[IBIS Ver]   3.2
[File Name]   sprm039d.ibs
[File Rev]   0.6
[Date]   April 12, 2004
[Source]   File Originated at Texas Instruments
[Disclaimer]   Please be aware that in the absence of a written agreement
|   Texas Instruments(TI) assumes no liability for:
|   (1) The accuracy of the IBIS models provided to your company
|   (2) The proper functioning of these Models in your design
|   or for any resulting applications;or
|   (3) Infringement of patents,copyrights, or intellectual
|   property rights resulting from your use of these models.
|   TI provides IBIS Models as a service to our customers and
|   therefore reserves the right to limit distribution of the
|   Models.
[Copyright]   Property of Texas Instruments Incorporated.
|   Unauthorized reproduction and/or distribution is strictly
|   prohibited.
|   This product is protected under copyright law and trade
|   secret law as an unpublished work.
|   Created 1999,(C) Copyright 1999-2000,
|   Texas Instruments Incorporated., All Rights Reserved.
|   These commodities are under the U.S.
|   Government distribution license control.As such,they are not
|   to be re-exported without the prior approval of the U.S.
|   Department of Commerce.
[Notes]   Includes new package and IO buffer models for 1.1 and 2.0.
|   REVISION HISTORY
|   Update for May 9, 2003 includes the following
|   -IO buffer name changes
|   -Addition of rising and falling waveforms to IO buffer models
|   -IBIS models generated using new SPICE simulations
|   -Updated package model
|   These new IBIS models (literature number srpm039c) are more accurate
|   than those posted before May 9, 2003. A simple evaluation (single
|   transmission line (50 ohm,500 pS delay) and single tranmission line (50
|   ohm, 500 pS delay) with a bifurcation) comparing the old IBIS models to the
|   new IBIS models was performed to provide a rough estimate of the
|   difference between the old and new models. The evaluation showed significant
|   differences may be observed in delay times for buffer models
|   describing the behavior of the McBSP, TIMER, UTOPIA, GPIO, PCI, and
|   EEPROM.  Only small differences were observed for EMIF buffers. Overall,
|   the delay times were smaller for the new IBIS models. We recommend that you
|   evaluate your design with the new models to determine any impact to your
|   system.
|   Update for April 12, 2004
|   The package model and IBIS models included in this file (sprm039d)
|   apply to TMS silicon for both silcon revision 1.1 and silicon
|   revision 2.0.
|   The package model and IBIS models included in sprm039d are unchanged
|   from those models provided in sprm039c.
[Component]   c6416_GLZ
[Manufacturer]   Texas Instruments
[Package]
|Variable   Typ   Min   Max
R_pkg		2.212e-01	1.101e-01	3.279e-01
L_pkg		4.011e-09	2.375e-09	5.798e-09
C_pkg		6.351e-13	3.910e-13	9.306e-13
[Pin] signal_name		model_name	R_pin		L_pin		C_pin
| Clock/PLL Configuration Section
   H4   CLKIN   IDH09_PE100   1.801e-01	3.100e-09	6.130e-13
  AE6	CLKOUT4_GP1	  IDH04_UOT335_PE100	2.381e-01	4.630e-09	6.473e-13
  AD6	CLKOUT6_GP2	  IDH04_UOT335_PE100	2.343e-01	3.341e-09	7.539e-13
   G1	  CLKMODE1   IDH04_PE100	2.962e-01	5.034e-09	7.789e-13
   H2	  CLKMODE0   IDH09_PE100   2.283e-01	3.995e-09	6.603e-13
| JTAG Emulation Section
 AB16   TMS   IDH09_PS100   1.377e-01	2.655e-09	4.925e-13
 AE19   TDO   IDH04_OUK83_PS100	2.511e-01	4.874e-09	6.498e-13
 AF18   TDI   IDH09_PS100   2.614e-01	5.224e-09	6.920e-13
 AF16   TCLK   IDH09_PS100   2.614e-01	5.224e-09	6.920e-13
 AB15   nTRST   IDH09_PE100   2.614e-01	5.224e-09	6.920e-13
 AE18   EMU9	  IDH04_UOT335_PS100	2.477e-01	4.401e-09	6.871e-13
 AC17   EMU8	  IDH04_UOT335_PS100	1.709e-01	3.536e-09	5.334e-13
 AF17   EMU7	  IDH04_UOT335_PS100	2.500e-01	5.062e-09	6.512e-13
 AD17   EMU6	  IDH04_UOT335_PS100	1.890e-01	3.826e-09	4.936e-13
 AE17   EMU5	  IDH04_UOT335_PS100	2.341e-01	4.430e-09	6.507e-13
 AC16   EMU4	  IDH04_UOT335_PS100	1.551e-01	2.968e-09	5.512e-13
 AD16   EMU3	  IDH04_UOT335_PS100	1.987e-01	3.671e-09	6.373e-13
 AE16   EMU2	  IDH04_UOT335_PS100	2.124e-01	3.853e-09	6.090e-13
 AC15   EMU1	  IDH04_UOT335_PS100	1.646e-01	3.085e-09	5.799e-13
 AF15   EMU0	  IDH04_UOT335_PS100	2.591e-01	4.625e-09	6.938e-13
 AC18   EMUCLK1	  IDH04_UOT335_PS100	1.860e-01	3.449e-09	5.618e-13
 AD18   EMUCLK0	  IDH04_UOT335_PS100	2.025e-01	3.878e-09	5.902e-13
| Resets, Interrupts, and General-Purpose IOs
  AC7   nRESET   IDH09	2.025e-01	3.878e-09	5.902e-13
   B4   NMI   IDH09_PE100   2.697e-01	4.485e-09	7.472e-13
  AF4	GP7_EXTINT7   IDH04_OUK83_PS100	2.697e-01	4.485e-09	7.472e-13
  AD5	GP6_EXTINT6   IDH04_OUK83_PS100	2.697e-01	4.485e-09	7.472e-13
  AE5	GP5_EXTINT5   IDH04_OUK83_PS100	2.697e-01	4.485e-09	7.472e-13
  AF5	GP4_EXTINT4   IDH04_OUK83_PS100	2.697e-01	4.485e-09	7.472e-13
   G3	GP15_nPRST   IDI01_OUG8B	2.697e-01	4.485e-09	7.472e-13
   F2	 GP14_PCLK   IDI01_OUG8B	2.546e-01	4.449e-09	7.097e-13
   G4	GP13_nPINTA   IDI01_OUG8B	2.546e-01	4.449e-09	7.097e-13
   J3	GP12_nPGNT   IDI01_OUG8B	2.546e-01	4.449e-09	7.097e-13
   F1	GP11_nPREQ   IDI01_OUG8B	2.546e-01	4.449e-09	7.097e-13
   L2	GP10_nPCBE3   IDI01_OUG8B	2.546e-01	4.449e-09	7.097e-13
   M3	GP9_PIDSEL   IDI01_OUG8B	1.917e-01	3.882e-09	5.354e-13
  AC6   GP3   IDH04_OUK83_PE100	1.851e-01	3.359e-09	6.075e-13
  AF6   GP0   IDH04_OUK83_PE100	2.922e-01	4.494e-09	8.253e-13
| Host-Port Interface (HPI) and Peripheral Component Interconnect (PCI)
  AA4   PCIEN   IDH09_PE100   2.922e-01	4.494e-09	8.253e-13
   R4	nHINT_nPFRAME   IDI01_OUG8B	2.922e-01	4.494e-09	8.253e-13
   R1	HCNTL1_nPDEVSEL   IDI01_OUG8B	2.602e-01	4.276e-09	7.238e-13
   T4	HCNTL0_nPSTOP   IDI01_OUG8B	1.544e-01	3.008e-09	5.439e-13
   R3	HHWIL_nPTRDY   IDI01_OUG8B	1.544e-01	3.008e-09	5.439e-13
   P1	HR/nW_nPCBE2   IDI01_OUG8B	1.544e-01	3.008e-09	5.439e-13
   T3	 nHAS_PPAR   IDI01_OUG8B	1.544e-01	3.008e-09	5.439e-13
   R2	nHCS_nPPERR   IDI01_OUG8B	1.544e-01	3.008e-09	5.439e-13
   T1	nHDS1_nPSERR   IDI01_OUG8B	1.544e-01	3.008e-09	5.439e-13
   T2	nHDS2_nPCBE1   IDI01_OUG8B	1.544e-01	3.008e-09	5.439e-13
   P4	nHRDY_nPIRDY   IDI01_OUG8B	1.432e-01	2.812e-09	4.868e-13
   J2	 HD31_AD31   IDI01_OUG8B	2.239e-01	3.881e-09	6.413e-13
   K3	 HD30_AD30   IDI01_OUG8B	2.011e-01	3.696e-09	5.567e-13
   J1	 HD29_AD29   IDI01_OUG8B	2.725e-01	4.920e-09	7.166e-13
   K4	 HD28_AD28   IDI01_OUG8B	1.590e-01	3.038e-09	5.268e-13
   K2	 HD27_AD27   IDI01_OUG8B	2.196e-01	4.083e-09	6.214e-13
   L3	 HD26_AD26   IDI01_OUG8B	1.822e-01	3.378e-09	5.755e-13
   K1	 HD25_AD25   IDI01_OUG8B	2.676e-01	5.238e-09	6.857e-13
   L4	 HD24_AD24   IDI01_OUG8B	1.692e-01	3.003e-09	5.620e-13
   L1	 HD23_AD23   IDI01_OUG8B	2.646e-01	4.791e-09	6.858e-13
   M4	 HD22_AD22   IDI01_OUG8B	1.455e-01	2.797e-09	5.032e-13
   M2	 HD21_AD21   IDI01_OUG8B	2.098e-01	3.830e-09	5.948e-13
   N4	 HD20_AD20   IDI01_OUG8B	1.611e-01	2.974e-09	5.102e-13
   M1	 HD19_AD19   IDI01_OUG8B	2.475e-01	4.493e-09	6.660e-13
   N5	 HD18_AD18   IDI01_OUG8B	1.114e-01	2.452e-09	4.378e-13
   N1	 HD17_AD17   IDI01_OUG8B	2.536e-01	4.462e-09	6.731e-13
   P5	 HD16_AD16   IDI01_OUG8B	1.387e-01	2.604e-09	5.119e-13
   U4	 HD15_AD15   IDI01_OUG8B	1.709e-01	3.367e-09	5.453e-13
   U1	 HD14_AD14   IDI01_OUG8B	2.504e-01	4.977e-09	6.598e-13
   U3	 HD13_AD13   IDI01_OUG8B	1.886e-01	3.777e-09	4.994e-13
   U2	 HD12_AD12   IDI01_OUG8B	2.321e-01	4.441e-09	6.047e-13
   V4	 HD11_AD11   IDI01_OUG8B	1.869e-01	3.381e-09	5.890e-13
   V1	 HD10_AD10   IDI01_OUG8B	2.598e-01	5.197e-09	6.873e-13
   V3	 HD09_AD09   IDI01_OUG8B	2.598e-01	5.197e-09	6.873e-13
   V2	 HD08_AD08   IDI01_OUG8B	2.598e-01	5.197e-09	6.873e-13
   W2	 HD07_AD07   IDI01_OUG8B	2.598e-01	5.197e-09	6.873e-13
   W4	 HD06_AD06   IDI01_OUG8B	2.598e-01	5.197e-09	6.873e-13
   Y1	 HD05_AD05   IDI01_OUG8B	2.598e-01	5.197e-09	6.873e-13
   Y3	 HD04_AD04   IDI01_OUG8B	2.598e-01	5.197e-09	6.873e-13
   Y2	 HD03_AD03   IDI01_OUG8B	2.598e-01	5.197e-09	6.873e-13
   Y4	 HD02_AD02   IDI01_OUG8B	2.598e-01	5.197e-09	6.873e-13
  AA1	 HD01_AD01   IDI01_OUG8B	2.598e-01	5.197e-09	6.873e-13
  AA3	 HD00_AD00   IDI01_OUG8B	2.598e-01	5.197e-09	6.873e-13
   W3   nPCBE0   IDI01_OUG8B	2.598e-01	5.197e-09	6.873e-13
  AD1   XSPCS   IDH04_OUK83_PE100	2.598e-01	5.197e-09	6.873e-13
| EMIF A Control Signals
  L26   nACE3	  IDH04_UOT335_PS100	2.598e-01	5.197e-09	6.873e-13
  K23   nACE2	  IDH04_UOT335_PS100	2.598e-01	5.197e-09	6.873e-13
  K24   nACE1	  IDH04_UOT335_PS100	2.598e-01	5.197e-09	6.873e-13
  K25   nACE0	  IDH04_UOT335_PS100	2.598e-01	5.197e-09	6.873e-13
  T23   nABE07	  IDH04_UOT335_PS100	2.598e-01	5.197e-09	6.873e-13
  T24   nABE06	  IDH04_UOT335_PS100	2.598e-01	5.197e-09	6.873e-13
  R25   nABE05	  IDH04_UOT335_PS100	2.598e-01	5.197e-09	6.873e-13
  R26   nABE04	  IDH04_UOT335_PS100	2.598e-01	5.197e-09	6.873e-13
  M25   nABE03	  IDH04_UOT335_PS100	2.598e-01	5.197e-09	6.873e-13
  M26   nABE02	  IDH04_UOT335_PS100	2.598e-01	5.197e-09	6.873e-13
  L23   nABE01	  IDH04_UOT335_PS100	2.598e-01	5.197e-09	6.873e-13
  L24   nABE00	  IDH04_UOT335_PS100	2.598e-01	5.197e-09	6.873e-13
  M22   nAPDT	  IDH04_UOT335_PS100	2.598e-01	5.197e-09	6.873e-13
| EMIF A Bus Arbitration
  N22   nAHOLDA	  IDH04_UOT335_PS100	2.598e-01	5.197e-09	6.873e-13
  V23   nAHOLD   IDH09_PS100   2.598e-01	5.197e-09	6.873e-13
  P22	  ABUSREQ0	  IDH04_UOT335_PS100	2.598e-01	5.197e-09	6.873e-13
| EMIF A Async/Sync Memory Control
  H25   AECLKIN   IDH09_PE100   2.511e-01	4.592e-09	6.768e-13
  J23	 AECLKOUT2	  IDH04_UOT335_PE100	1.851e-01	3.434e-09	5.608e-13
  J26	 AECLKOUT1	  IDH04_UOT335_PE100	2.599e-01	5.229e-09	6.780e-13
  J25   nASDCAS	  IDH04_UOT335_PS100	2.467e-01	4.341e-09	6.879e-13
  J24   nASDRAS	  IDH04_UOT335_PS100	2.014e-01	3.844e-09	5.854e-13
  K26   nASDWE	  IDH04_UOT335_PS100	2.494e-01	5.112e-09	6.385e-13
  L25   ASDCKE	  IDH04_UOT335_PS100	2.118e-01	3.884e-09	5.955e-13
  R22   nASOE3	  IDH04_UOT335_PS100	2.118e-01	3.884e-09	5.955e-13
  L22   AARDY   IDH09_PS100   1.370e-01	2.710e-09	4.841e-13
| EMIF A Address
  T22   AEA22	  IDH04_UOT335_PE100	1.229e-01	2.684e-09	4.276e-13
  V24   AEA21	  IDH04_UOT335_PE100	2.064e-01	3.768e-09	6.312e-13
  V25   AEA20	  IDH04_UOT335_PE100	2.195e-01	4.186e-09	6.132e-13
  V26   AEA19	  IDH04_UOT335_PE100	2.732e-01	4.782e-09	7.055e-13
  U23   AEA18	  IDH04_UOT335_PE100	1.584e-01	2.852e-09	5.393e-13
  U24   AEA17	  IDH04_UOT335_PE100	2.008e-01	3.829e-09	5.212e-13
  U25   AEA16	  IDH04_UOT335_PE100	2.141e-01	4.207e-09	5.706e-13
  U26   AEA15	  IDH04_UOT335_PE100	2.663e-01	5.219e-09	6.884e-13
  T25   AEA14	  IDH04_UOT335_PE100	2.291e-01	3.977e-09	6.514e-13
  T26   AEA13	  IDH04_UOT335_PE100	2.614e-01	4.919e-09	6.730e-13
  R23   AEA12	  IDH04_UOT335_PE100	1.480e-01	3.031e-09	5.090e-13
  R24   AEA11	  IDH04_UOT335_PE100	1.952e-01	3.745e-09	6.090e-13
  P23   AEA10	  IDH04_UOT335_PE100	1.599e-01	3.076e-09	4.973e-13
  P24   AEA09	  IDH04_UOT335_PE100	1.599e-01	3.076e-09	4.973e-13
  P26   AEA08	  IDH04_UOT335_PE100	1.599e-01	3.076e-09	4.973e-13
  N23   AEA07	  IDH04_UOT335_PE100	1.599e-01	3.076e-09	4.973e-13
  N24   AEA06	  IDH04_UOT335_PE100	1.599e-01	3.076e-09	4.973e-13
  N26   AEA05	  IDH04_UOT335_PE100	1.599e-01	3.076e-09	4.973e-13
  M23   AEA04	  IDH04_UOT335_PE100	1.599e-01	3.076e-09	4.973e-13
  M24   AEA03	  IDH04_UOT335_PE100	1.599e-01	3.076e-09	4.973e-13
| EMIF A Data
 AF24   AED63	  IDH04_UOT335_PS100	3.137e-01	4.620e-09	8.662e-13
 AF23   AED62	  IDH04_UOT335_PS100	3.279e-01	4.771e-09	9.306e-13
 AE23   AED61	  IDH04_UOT335_PS100	2.711e-01	4.106e-09	8.091e-13
 AE22   AED60	  IDH04_UOT335_PS100	2.891e-01	4.209e-09	8.615e-13
 AD22   AED59	  IDH04_UOT335_PS100	2.423e-01	3.976e-09	6.864e-13
 AF22   AED58	  IDH04_UOT335_PS100	2.977e-01	4.773e-09	8.420e-13
 AD21   AED57	  IDH04_UOT335_PS100	2.300e-01	3.370e-09	7.485e-13
 AE21   AED56	  IDH04_UOT335_PS100	2.753e-01	4.129e-09	8.309e-13
 AC21   AED55	  IDH04_UOT335_PS100	2.164e-01	3.287e-09	6.853e-13
 AF21   AED54	  IDH04_UOT335_PS100	2.835e-01	5.063e-09	7.235e-13
 AD20   AED53	  IDH04_UOT335_PS100	2.224e-01	4.053e-09	6.338e-13
 AE20   AED52	  IDH04_UOT335_PS100	2.582e-01	4.676e-09	6.914e-13
 AC20   AED51	  IDH04_UOT335_PS100	2.074e-01	3.082e-09	7.302e-13
 AF20   AED50	  IDH04_UOT335_PS100	2.708e-01	4.795e-09	7.375e-13
 AC19   AED49	  IDH04_UOT335_PS100	1.905e-01	3.252e-09	6.365e-13
 AD19   AED48	  IDH04_UOT335_PS100	2.081e-01	3.848e-09	5.927e-13
  W24   AED47	  IDH04_UOT335_PS100	2.123e-01	3.951e-09	6.323e-13
  W23   AED46	  IDH04_UOT335_PS100	1.710e-01	3.189e-09	5.673e-13
  Y26   AED45	  IDH04_UOT335_PS100	2.823e-01	4.619e-09	7.521e-13
  Y23   AED44	  IDH04_UOT335_PS100	1.758e-01	3.461e-09	5.750e-13
  Y25   AED43	  IDH04_UOT335_PS100	2.336e-01	4.207e-09	6.577e-13
  Y24   AED42	  IDH04_UOT335_PS100	2.187e-01	3.908e-09	6.476e-13
 AA26   AED41	  IDH04_UOT335_PS100	2.881e-01	5.195e-09	7.377e-13
 AA23   AED40	  IDH04_UOT335_PS100	1.857e-01	3.342e-09	6.147e-13
 AA25   AED39	  IDH04_UOT335_PS100	2.386e-01	4.607e-09	6.579e-13
 AA24   AED38	  IDH04_UOT335_PS100	2.252e-01	4.506e-09	5.857e-13
 AB26   AED37	  IDH04_UOT335_PS100	3.007e-01	5.253e-09	7.746e-13
 AB24   AED36	  IDH04_UOT335_PS100	2.392e-01	4.041e-09	6.955e-13
 AB25   AED35	  IDH04_UOT335_PS100	2.521e-01	4.603e-09	6.570e-13
 AC25   AED34	  IDH04_UOT335_PS100	2.807e-01	4.863e-09	7.510e-13
 AC26   AED33	  IDH04_UOT335_PS100	2.960e-01	5.121e-09	7.683e-13
 AD26   AED32	  IDH04_UOT335_PS100	3.008e-01	4.916e-09	8.215e-13
  C26   AED31	  IDH04_UOT335_PS100	3.097e-01	5.406e-09	7.617e-13
  D26   AED30	  IDH04_UOT335_PS100	3.225e-01	5.517e-09	8.165e-13
  D25   AED29	  IDH04_UOT335_PS100	2.683e-01	4.604e-09	7.287e-13
  E25   AED28	  IDH04_UOT335_PS100	2.825e-01	4.968e-09	7.318e-13
  E24   AED27	  IDH04_UOT335_PS100	2.414e-01	4.280e-09	6.457e-13
  E26   AED26	  IDH04_UOT335_PS100	2.953e-01	5.146e-09	7.737e-13
  F24   AED25	  IDH04_UOT335_PS100	2.271e-01	4.100e-09	5.755e-13
  F25   AED24	  IDH04_UOT335_PS100	2.711e-01	4.743e-09	7.222e-13
  F23   AED23	  IDH04_UOT335_PS100	2.131e-01	3.580e-09	6.337e-13
  F26   AED22	  IDH04_UOT335_PS100	2.841e-01	5.079e-09	7.359e-13
  G24   AED21	  IDH04_UOT335_PS100	2.217e-01	4.037e-09	6.338e-13
  G25   AED20	  IDH04_UOT335_PS100	2.556e-01	4.841e-09	6.769e-13
  G23   AED19	  IDH04_UOT335_PS100	2.034e-01	3.544e-09	6.297e-13
  G26   AED18	  IDH04_UOT335_PS100	2.698e-01	4.780e-09	7.327e-13
  H23   AED17	  IDH04_UOT335_PS100	1.904e-01	3.427e-09	5.839e-13
  H24   AED16	  IDH04_UOT335_PS100	2.066e-01	3.899e-09	5.834e-13
  C19   AED15	  IDH04_UOT335_PS100	2.140e-01	3.969e-09	6.377e-13
  D19   AED14	  IDH04_UOT335_PS100	1.703e-01	3.235e-09	5.662e-13
  A20   AED13	  IDH04_UOT335_PS100	2.811e-01	4.710e-09	7.445e-13
  D20   AED12	  IDH04_UOT335_PS100	1.756e-01	3.477e-09	5.767e-13
  B20   AED11	  IDH04_UOT335_PS100	2.338e-01	4.170e-09	6.537e-13
  C20   AED10	  IDH04_UOT335_PS100	2.189e-01	3.889e-09	6.502e-13
  A21   AED09	  IDH04_UOT335_PS100	2.189e-01	3.889e-09	6.502e-13
  D21   AED08	  IDH04_UOT335_PS100	2.189e-01	3.889e-09	6.502e-13
  B21   AED07	  IDH04_UOT335_PS100	2.189e-01	3.889e-09	6.502e-13
  C21   AED06	  IDH04_UOT335_PS100	2.189e-01	3.889e-09	6.502e-13
  A22   AED05	  IDH04_UOT335_PS100	2.189e-01	3.889e-09	6.502e-13
  C22   AED04	  IDH04_UOT335_PS100	2.189e-01	3.889e-09	6.502e-13
  B22   AED03	  IDH04_UOT335_PS100	2.189e-01	3.889e-09	6.502e-13
  B23   AED02	  IDH04_UOT335_PS100	2.189e-01	3.889e-09	6.502e-13
  A23   AED01	  IDH04_UOT335_PS100	2.189e-01	3.889e-09	6.502e-13
  A24   AED00	  IDH04_UOT335_PS100	2.189e-01	3.889e-09	6.502e-13
| EMIF B Control Signals
  A13   nBCE3	  IDH04_UOT335_PS100	2.189e-01	3.889e-09	6.502e-13
  C12   nBCE2	  IDH04_UOT335_PS100	2.189e-01	3.889e-09	6.502e-13
  B12   nBCE1	  IDH04_UOT335_PS100	2.189e-01	3.889e-09	6.502e-13
  A12   nBCE0	  IDH04_UOT335_PS100	2.189e-01	3.889e-09	6.502e-13
  D13   nBBE01	  IDH04_UOT335_PS100	2.189e-01	3.889e-09	6.502e-13
  C13   nBBE00	  IDH04_UOT335_PS100	2.189e-01	3.889e-09	6.502e-13
  E12   nBPDT	  IDH04_UOT335_PS100	2.189e-01	3.889e-09	6.502e-13
| EMIF B Bus Arbitration
  E13   nBHOLDA	  IDH04_UOT335_PS100	2.189e-01	3.889e-09	6.502e-13
  B19   nBHOLD   IDH09_PS100   2.189e-01	3.889e-09	6.502e-13
  E14	  BBUSREQ0	  IDH04_UOT335_PS100	2.189e-01	3.889e-09	6.502e-13
| EMIF B Async/Sync Memory Control
  A11   BECLKIN   IDH09_PE100   2.464e-01	4.786e-09	6.528e-13
  D11	 BECLKOUT2	  IDH04_UOT335_PE100	1.551e-01	3.003e-09	5.234e-13
  D12	 BECLKOUT1	  IDH04_UOT335_PE100	1.654e-01	3.214e-09	5.248e-13
  A10   nBSDCAS	  IDH04_UOT335_PS100	2.586e-01	5.225e-09	6.597e-13
  B11   nBSDRAS	  IDH04_UOT335_PS100	2.119e-01	3.872e-09	5.932e-13
  C11   nBSDWE	  IDH04_UOT335_PS100	1.986e-01	3.667e-09	5.913e-13
  E15   nBSOE3	  IDH04_UOT335_PS100	1.986e-01	3.667e-09	5.913e-13
  E11   BARDY   IDH09   1.365e-01	2.770e-09	4.880e-13
| EMIF B Address
  E16   BEA20	  IDH04_UOT335_PS100	1.226e-01	2.604e-09	4.665e-13
  D18   BEA19	  IDH04_UOT335_PS100	1.641e-01	2.969e-09	5.594e-13
  C18   BEA18	  IDH04_UOT335_PE100	2.067e-01	3.758e-09	6.201e-13
  B18   BEA17	  IDH04_UOT335_PE100	2.194e-01	4.208e-09	6.099e-13
  A18   BEA16	  IDH04_UOT335_PE100	2.767e-01	5.325e-09	6.838e-13
  D17   BEA15	  IDH04_UOT335_PE100	1.577e-01	2.912e-09	5.360e-13
  C17   BEA14	  IDH04_UOT335_PE100	2.010e-01	3.803e-09	5.328e-13
  B17   BEA13	  IDH04_UOT335_PE100	2.141e-01	4.201e-09	5.714e-13
  A17   BEA12	  IDH04_UOT335_PE100	2.663e-01	5.209e-09	6.868e-13
  D16   BEA11	  IDH04_UOT335_PE100	1.659e-01	3.222e-09	5.785e-13
  C16   BEA10	  IDH04_UOT335_PE100	1.798e-01	3.385e-09	6.098e-13
  B16   BEA09	  IDH04_UOT335_PE100	1.798e-01	3.385e-09	6.098e-13
  A16   BEA08	  IDH04_UOT335_PE100	1.798e-01	3.385e-09	6.098e-13
  D15   BEA07	  IDH04_UOT335_PE100	1.798e-01	3.385e-09	6.098e-13
  C15   BEA06	  IDH04_UOT335_PE100	1.798e-01	3.385e-09	6.098e-13
  B15   BEA05	  IDH04_UOT335_PE100	1.798e-01	3.385e-09	6.098e-13
  A15   BEA04	  IDH04_UOT335_PE100	1.798e-01	3.385e-09	6.098e-13
  D14   BEA03	  IDH04_UOT335_PE100	1.798e-01	3.385e-09	6.098e-13
  C14   BEA02	  IDH04_UOT335_PE100	1.798e-01	3.385e-09	6.098e-13
  A14   BEA01	  IDH04_UOT335_PE100	1.798e-01	3.385e-09	6.098e-13
| EMIF B Data
   D7   BED15	  IDH04_UOT335_PS100	2.025e-01	3.629e-09	6.353e-13
   B6   BED14	  IDH04_UOT335_PS100	2.713e-01	4.736e-09	7.195e-13
   C7   BED13	  IDH04_UOT335_PS100	2.210e-01	4.136e-09	6.396e-13
   A6   BED12	  IDH04_UOT335_PS100	2.839e-01	5.035e-09	7.333e-13
   D8   BED11	  IDH04_UOT335_PS100	1.903e-01	3.261e-09	6.403e-13
   B7   BED10	  IDH04_UOT335_PS100	2.577e-01	4.650e-09	6.879e-13
   C8   BED09	  IDH04_UOT335_PS100	2.577e-01	4.650e-09	6.879e-13
   A7   BED08	  IDH04_UOT335_PS100	2.577e-01	4.650e-09	6.879e-13
   C9   BED07	  IDH04_UOT335_PS100	2.577e-01	4.650e-09	6.879e-13
   B8   BED06	  IDH04_UOT335_PS100	2.577e-01	4.650e-09	6.879e-13
   D9   BED05	  IDH04_UOT335_PS100	2.577e-01	4.650e-09	6.879e-13
   B9   BED04	  IDH04_UOT335_PS100	2.577e-01	4.650e-09	6.879e-13
  C10   BED03	  IDH04_UOT335_PS100	2.577e-01	4.650e-09	6.879e-13
   A9   BED02	  IDH04_UOT335_PS100	2.577e-01	4.650e-09	6.879e-13
  D10   BED01	  IDH04_UOT335_PS100	2.577e-01	4.650e-09	6.879e-13
  B10   BED00	  IDH04_UOT335_PS100	2.577e-01	4.650e-09	6.879e-13
| Timer 2
   A4   TOUT2   IDH04_OUK83_PE100	3.211e-01	5.798e-09	7.928e-13
   C5   TINP2   IDH09_PE100   2.423e-01	4.149e-09	6.777e-13
| Timer 1
   B5   TOUT1   IDH04_OUK83_PE100	2.850e-01	4.720e-09	7.582e-13
   A5   TINP1   IDH09_PE100   2.956e-01	5.023e-09	7.720e-13
| Timer 0
   D6   TOUT0   IDH04_OUK83_PE100	2.113e-01	3.835e-09	6.281e-13
   C6   TINP0   IDH09_PE100   2.266e-01	4.066e-09	6.171e-13
| MultiChannel Buffered Serial Port 2 (McBSP2)
  AF3	 MCBSP2_EN   IDH09_PE100   3.053e-01	4.791e-09	8.195e-13
  AE4	 CLKS2_GP8   IDH04_OUK83_PE100	2.815e-01	4.759e-09	7.525e-13
  AB1   CLKR2   IDH04_OUK83_PE100	2.952e-01	5.337e-09	7.495e-13
  AC2	CLKX2_XSPCLK   IDH04_OUK83_PE100	2.690e-01	4.510e-09	7.463e-13
  AB3	 DR2_XSPDI   IDH04_PS100	2.430e-01	4.177e-09	6.584e-13
  AA2	 DX2_XSPDO   IDH04_OUK83_PS100	2.703e-01	4.736e-09	7.142e-13
  AC1   FSR2   IDH04_OUK83_PE100	3.209e-01	5.708e-09	7.989e-13
  AB2   FSX2   IDH04_OUK83_PE100	2.854e-01	4.677e-09	7.645e-13
| MultiChannel Buffered Serial Port 1 (McBSP1)
  AC8	CLKS1_URADDR3   IDH04_OUK83	1.696e-01	3.371e-09	5.336e-13
 AC10	CLKR1_URADDR2   IDH04_OUK83	1.577e-01	2.917e-09	5.345e-13
 AB12	CLKX1_URADDR4   IDH04_OUK83	1.314e-01	2.568e-09	4.920e-13
 AF11	DR1_UXADDR1   IDH04_OUK83	2.619e-01	4.872e-09	6.818e-13
 AB11	DX1_UXADDR4   IDH04_OUK83	1.224e-01	2.641e-09	4.477e-13
  AC9	FSR1_UXADDR2   IDH04_OUK83	1.641e-01	2.958e-09	5.482e-13
 AB13	FSX1_UXADDR3   IDH04_OUK83	1.112e-01	2.390e-09	4.431e-13
| MultiChannel Buffered Serial Port 0 (McBSP0)
   F4   CLKS0   IDH09_PE100   1.913e-01	3.477e-09	6.149e-13
   D1   CLKR0   IDH04_OUK83_PE100	2.976e-01	5.157e-09	7.602e-13
   E1   CLKX0   IDH04_OUK83_PE100	3.080e-01	5.297e-09	7.859e-13
   D2   DR0   IDH04_PS100	2.825e-01	4.838e-09	7.380e-13
   E2   DX0   IDH04_OUK83_PS100	2.580e-01	4.588e-09	6.760e-13
   C1   FSR0   IDH04_OUK83_PE100	3.009e-01	4.906e-09	7.948e-13
   E3   FSX0   IDH04_OUK83_PE100	2.445e-01	4.090e-09	6.962e-13
| UTOPIA Transmit Interface
 AD11   UXCLK   IDH09	1.796e-01	3.416e-09	5.747e-13
 AC14   UXCLAV   IDH04_OUK83	1.451e-01	2.709e-09	4.991e-13
 AE15   nUXENB   IDH04_OUK83	1.451e-01	2.709e-09	4.991e-13
 AC13   UXSOC   IDH04_OUK83	1.609e-01	2.896e-09	5.178e-13
  AE9   UXADDR0   IDH04_OUK83	2.212e-01	4.035e-09	6.442e-13
 AD10   UXDATA7   IDH04_OUK83	2.009e-01	3.820e-09	5.217e-13
  AD9   UXDATA6   IDH04_OUK83	2.069e-01	3.735e-09	6.102e-13
  AD8   UXDATA5   IDH04_OUK83	2.137e-01	4.020e-09	6.080e-13
  AE8   UXDATA4   IDH04_OUK83	2.278e-01	4.253e-09	6.349e-13
  AF9   UXDATA3   IDH04_OUK83	2.793e-01	5.310e-09	6.864e-13
  AF7   UXDATA2   IDH04_OUK83	2.810e-01	4.704e-09	7.582e-13
  AE7   UXDATA1   IDH04_OUK83	2.331e-01	4.270e-09	6.513e-13
  AD7   UXDATA0   IDH04_OUK83	2.198e-01	3.771e-09	6.554e-13
| UTOPIA Receive Interface
 AD12   URCLK   IDH09	1.922e-01	3.803e-09	5.427e-13
 AF14   URCLAV   IDH04_OUK83	2.495e-01	4.260e-09	6.591e-13
 AD15   nURENB   IDH04_OUK83	2.495e-01	4.260e-09	6.591e-13
 AB14   URSOC   IDH04	1.337e-01	2.442e-09	4.893e-13
 AF10   URADDR1   IDH04_OUK83	2.663e-01	5.227e-09	6.845e-13
 AE10   URADDR0   IDH04_OUK83	2.146e-01	4.151e-09	5.705e-13
 AF12   URDATA7   IDH04	2.456e-01	4.323e-09	6.794e-13
 AE11   URDATA6   IDH04	2.291e-01	4.061e-09	6.408e-13
 AF13   URDATA5   IDH04	2.560e-01	4.376e-09	6.811e-13
 AC11   URDATA4   IDH04	1.656e-01	3.268e-09	5.357e-13
 AC12   URDATA3   IDH04	1.441e-01	3.075e-09	4.975e-13
 AE12   URDATA2   IDH04	2.104e-01	3.651e-09	6.043e-13
 AD14   URDATA1   IDH04	1.921e-01	3.213e-09	5.935e-13
 AD13   URDATA0   IDH04	1.677e-01	5.324e-09	3.910e-13
| End of Package Model
[Component]   IDH04_PE100
[Manufacturer]   Texas Instruments
[Package]
|   typ   min   max
R_pkg   0   0   0
L_pkg   0   0   0
C_pkg   0   0   0
[Pin]   signal_name   model_name   R_pin   L_pin   C_pin
   1   A   IDH04_PE100   0   0   0
[Component]   IDH04_UOT335_PE100
[Manufacturer]   Texas Instruments
[Package]
|   typ   min   max
R_pkg   0   0   0
L_pkg   0   0   0
C_pkg   0   0   0
[Pin]   signal_name   model_name   R_pin   L_pin   C_pin
   1   Y  IDH04_UOT335_PE100   0   0   0
[Component]   IDH04_PS100
[Manufacturer]   Texas Instruments
[Package]
|   typ   min   max
R_pkg   0   0   0
L_pkg   0   0   0
C_pkg   0   0   0
[Pin]   signal_name   model_name   R_pin   L_pin   C_pin
   1   A   IDH04_PS100   0   0   0
[Component]   IDH04_OUK83_PS100
[Manufacturer]   Texas Instruments
[Package]
|   typ   min   max
R_pkg   0   0   0
L_pkg   0   0   0
C_pkg   0   0   0
[Pin]   signal_name   model_name   R_pin   L_pin   C_pin
   1   Y   IDH04_OUK83_PS100   0   0   0
[Component]   IDH04_UOT335_PS100
[Manufacturer]   Texas Instruments
[Package]
|   typ   min   max
R_pkg   0   0   0
L_pkg   0   0   0
C_pkg   0   0   0
[Pin]   signal_name   model_name   R_pin   L_pin   C_pin
   1   Y  IDH04_UOT335_PS100   0   0   0
[Component]   IDH09
[Manufacturer]   Texas Instruments
[Package]
|   typ   min   max
R_pkg   0   0   0
L_pkg   0   0   0
C_pkg   0   0   0
[Pin]   signal_name   model_name   R_pin   L_pin   C_pin
   1   A   IDH09   0   0   0
[Component]   IDH09_PS100
[Manufacturer]   Texas Instruments
[Package]
|   typ   min   max
R_pkg   0   0   0
L_pkg   0   0   0
C_pkg   0   0   0
[Pin]   signal_name   model_name   R_pin   L_pin   C_pin
   1   A   IDH09_PS100   0   0   0
[Component]   IDH09_PE100
[Manufacturer]   Texas Instruments
[Package]
|   typ   min   max
R_pkg   0   0   0
L_pkg   0   0   0
C_pkg   0   0   0
[Pin]   signal_name   model_name   R_pin   L_pin   C_pin
   1   A   IDH09_PE100   0   0   0
[Component]   IDI01_OUG8B
[Manufacturer]   Texas Instruments
[Package]
|   typ   min   max
R_pkg   0   0   0
L_pkg   0   0   0
C_pkg   0   0   0
[Pin]   signal_name   model_name   R_pin   L_pin   C_pin
   1   Y   IDI01_OUG8B   0   0   0
[Component]   IDH04_OUK83_PE100
[Manufacturer]   Texas Instruments
[Package]
|   typ   min   max
R_pkg   0   0   0
L_pkg   0   0   0
C_pkg   0   0   0
[Pin]   signal_name   model_name   R_pin   L_pin   C_pin
   1   Y   IDH04_OUK83_PE100   0   0   0
[Component]   IDH04_OUK83
[Manufacturer]   Texas Instruments
[Package]
|   typ   min   max
R_pkg   0   0   0
L_pkg   0   0   0
C_pkg   0   0   0
[Pin]   signal_name   model_name   R_pin   L_pin   C_pin
   1   Y   IDH04_OUK83   0   0   0
[Component]   IDH04
[Manufacturer]   Texas Instruments
[Package]
|   typ   min   max
R_pkg   0   0   0
L_pkg   0   0   0
C_pkg   0   0   0
[Pin]   signal_name   model_name   R_pin   L_pin   C_pin
   1   A   IDH04   0   0   0
| Models and submodels in the file (12): IDH04_PE100 (Input), IDH04_UOT335_PE100 (I/O), IDH04_PS100 (Input), IDH04_OUK83_PS100 (I/O), IDH04_UOT335_PS100 (I/O), IDH09 (Input), IDH09_PS100 (Input), IDH09_PE100 (Input), IDI01_OUG8B (I/O), IDH04_OUK83_PE100 (I/O), IDH04_OUK83 (I/O), IDH04 (Input)
